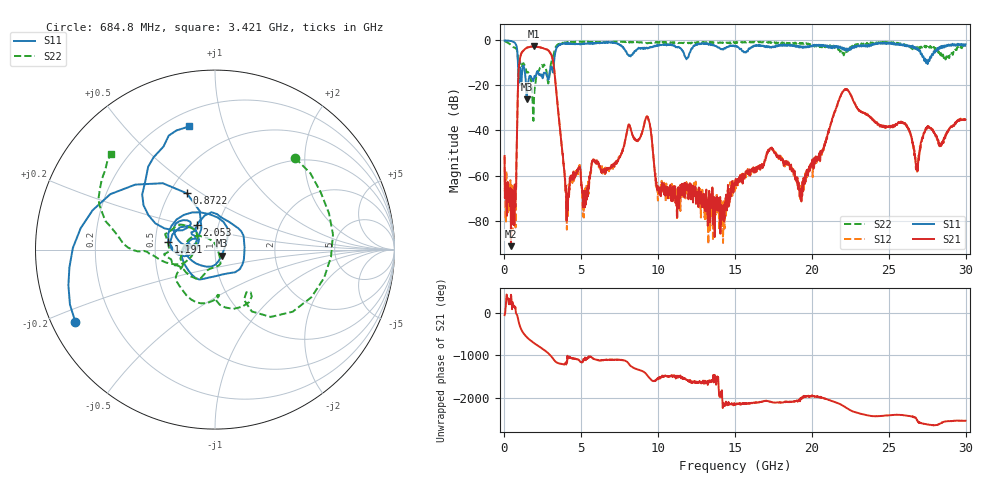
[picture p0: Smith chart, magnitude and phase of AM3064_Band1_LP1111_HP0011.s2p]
# Hz S DB R 50.0
!freq dBS11 angS11 dBS21 angS21 dBS12 angS12 dBS22 angS22
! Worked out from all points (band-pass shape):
!   1600 points, 10 MHz to 29.98 GHz, reference 50 ohm
!   highest |S21| = -2.70 dB at 1.922 GHz (marker M1); lowest = -91.4 dB at 422.4 MHz (marker M2)
!   |S21| within 3 dB of the highest: 1.101 GHz to 2.989 GHz (1.888 GHz wide, 92.3 % of centre)
!   lowest |S11| = -26.1 dB at 1.453 GHz (marker M3), VSWR 1.10, Z = 53.6 - j3.59 ohm
!   |S11| at or under -10 dB: 876.9 MHz to 3.219 GHz (2.342 GHz wide, 114 % of centre); 27.4213 GHz to 27.43624 GHz (14.94 MHz wide, 0.0545 % of centre); 27.51058 GHz to 27.55259 GHz (42.01 MHz wide, 0.153 % of centre)
!   |S22| runs from -35.7 to -0.2 dB; largest |S21 - S12| = 0.01
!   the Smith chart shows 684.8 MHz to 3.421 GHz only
!   S11 on the Smith chart (normalised r, x): 684.8 MHz: 0.07, -0.24; 872.2 MHz: 0.61, +0.44; 1.191 GHz: 0.59, +0.06; 2.053 GHz: 0.79, +0.22; 3.421 GHz: 0.29, +0.77
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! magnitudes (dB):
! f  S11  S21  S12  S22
! 10 MHz  -0.1  -51.3  -51.7  -0.2
! 422.4 MHz  -0.3  -91.4  -73.3  -2.1
! 684.8 MHz  -1.2  -72.3  -66.3  -3.4
! 872.2 MHz  -9.1  -22.6  -22.6  -7.9
! 1.191 GHz  -11.6  -4.9  -4.8  -10.4
! 1.453 GHz  -26.1  -3.3  -3.2  -14.3
! 1.922 GHz  -16.8  -2.7  -2.7  -25.8
! 2.053 GHz  -15.5  -2.8  -2.7  -16.8
! 3.028 GHz  -11.7  -6.2  -6.1  -10.2
! 3.421 GHz  -3.1  -26.4  -26.3  -2.1
! 4.077 GHz  -1.4  -76.2  -72.3  -0.8
! 5.015 GHz  -1.5  -64.1  -63.9  -0.5
! 9.269 GHz  -3.2  -33.9  -33.7  -1.3
! 10 GHz  -2.2  -66.0  -64.7  -0.9
! 14.2 GHz  -4.0  -75.5  -82.6  -0.9
! 15 GHz  -2.6  -64.3  -64.9  -1.3
! 17.31 GHz  -3.0  -47.8  -47.6  -0.9
! 19.99 GHz  -2.7  -54.5  -55.8  -1.8
! 22.13 GHz  -4.3  -22.0  -22.1  -5.3
! 25 GHz  -1.0  -38.4  -38.5  -1.0
! 26.81 GHz  -3.6  -56.2  -56.3  -3.7
! 29.98 GHz  -1.8  -35.2  -35.4  -2.8
